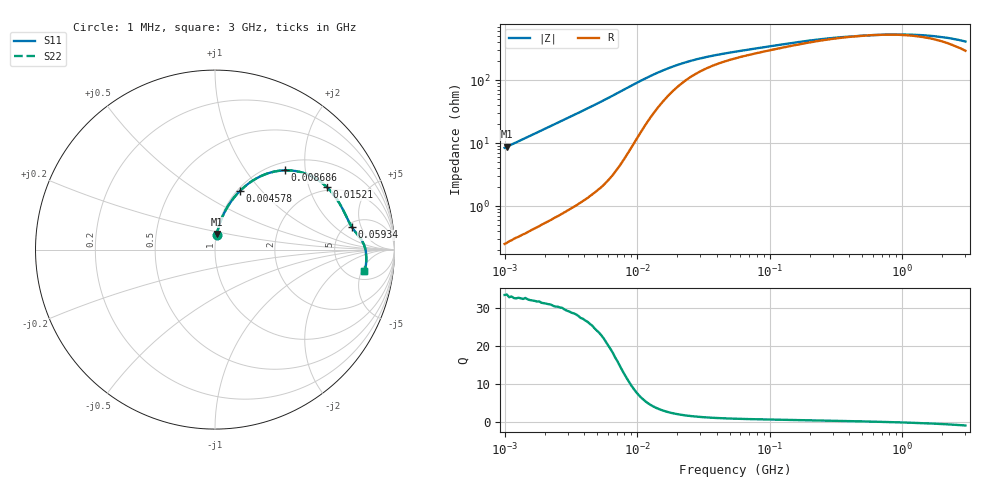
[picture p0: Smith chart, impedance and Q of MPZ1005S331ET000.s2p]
! S-Parameter Data Generated by TDK Corporation
! Copyright(C) 2025 TDK Corporation.
! All Rights Reserved.
! TDK P/N: MPZ1005S331ET000 (Chip Bead)
! Property: |Z|=330ohm at 100MHz
! Size(LxWxT): 1x0.5x0.5mm
! Model Type: s2p (Touchstone File Format Version 1.0)
! Frequency: DC=Yes Start=1MHz Stop=3000MHz 202points Log-sweep
! Model Generated on Feb. 6, 2025
! Terms and conditions regarding TDK Simulation Models:
! 1)This simulation model is being provided solely for informational
!  purposes. Please refer to the specifications of the products in
!  terms of detailed characteristics of such products.
! 2)In no event shall TDK Corporation of any of its subsidiaries be
!  liable for any loss or damage arising, directly or indirectly,
!  from any information contained in this simulation model, including,
!  but not limited to loss or damages arising from any inaccuracies,
!  omissions or errors in connection with such information.
! 3)Any and all copyrights on this simulation model are owned by
!  TDK Corporation.  Duplication or redistribution of this simulation
!  model without prior written permission from TDK Corporation
!  is prohibited.
! 4)This simulation model is subject to any modification or change
!  without any prior notice.
! 5)Neither TDK Corporation nor any of its subsidiaries shall make any
!  warranty, express or implied, including but not limited to the
!  correctness, implied warranties of merchantability and fitness for
!  a particular purpose with respect to this simulation models.
! 6)The use of this simulation model shall be deemed to have consented
!  to the terms and conditions hereof.
! Port Assignments:
!  1 ---@@@--- 2
! Applicable Conditions:
!  Temperature = 25 degC
!  DC Bias Current = 0 A
!  Small Signal Operation
# Hz S MA R 50
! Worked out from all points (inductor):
!   201 points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, 1 MHz to 3 GHz, reference 50 ohm
!   read as one part in series: L = 1.34 uH near 1.041 MHz
!   highest Q = 33.4 at 1.041 MHz (marker M1), where L = 1.34 uH
!   self-resonance near 647.5 MHz
!   S11 on the Smith chart (normalised r, x): 1 MHz: 1.01, +0.17; 4.578 MHz: 1.03, +0.77; 8.686 MHz: 1.15, +1.55; 15.21 MHz: 1.85, +2.64; 59.34 MHz: 5.60, +3.48; 3 GHz: 6.82, -5.70
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1000000  0.08366 83.5  0.994 -4.8  0.994 -4.8  0.08366 83.5
1040844  0.08707 83.3  0.9936 -5.0  0.9936 -5.0  0.08707 83.3
2226959  0.1819 77.7  0.9774 -10.5  0.9774 -10.5  0.1819 77.7
3900413  0.3076 70.0  0.9402 -17.9  0.9402 -17.9  0.3076 70.0
4577760  0.3553 66.9  0.9208 -20.8  0.9208 -20.8  0.3553 66.9
6305767  0.4671 59.2  0.8601 -27.8  0.8601 -27.8  0.4671 59.2
8686058  0.5874 48.8  0.7553 -35.8  0.7553 -35.8  0.5874 48.8
1.104425e7  0.6589 39.9  0.6508 -40.5  0.6508 -40.5  0.6589 39.9
1.461624e7  0.7086 30.5  0.5306 -42.7  0.5306 -42.7  0.7086 30.5
1.521322e7  0.7133 29.4  0.5151 -42.7  0.5151 -42.7  0.7133 29.4
1.934349e7  0.7329 23.2  0.4352 -41.5  0.4352 -41.5  0.7329 23.2
2.664524e7  0.7474 17.1  0.3608 -37.6  0.3608 -37.6  0.7474 17.1
3.670325e7  0.7577 13.1  0.3133 -33.2  0.3133 -33.2  0.7577 13.1
5.477226e7  0.7704 9.8  0.2743 -28.6  0.2743 -28.6  0.7704 9.8
5.933785e7  0.7732 9.3  0.2679 -27.8  0.2679 -27.8  0.7732 9.3
2.136344e8  0.8187 3.7  0.1905 -16.2  0.1905 -16.2  0.8187 3.7
4.0536e8  0.8323 1.6  0.1696 -7.6  0.1696 -7.6  0.8323 1.6
8.005644e8  0.8407 -0.8  0.1598 4.1  0.1598 4.1  0.8407 -0.8
1.194682e9  0.8434 -2.4  0.1614 12.9  0.1614 12.9  0.8434 -2.4
1.712864e9  0.845 -4.3  0.1697 21.9  0.1697 21.9  0.845 -4.3
2.266846e9  0.8452 -6.1  0.1831 29.4  0.1831 29.4  0.8452 -6.1
3e9  0.8418 -8.3  0.2067 36.1  0.2067 36.1  0.8418 -8.3
